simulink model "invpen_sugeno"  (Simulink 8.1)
settings: Solver=ode5  SolverMode=SingleTasking  StartTime=0.0  StopTime=1000  FixedStep=.01  MaxStep=0.1  RelTol=1e-3  AbsTol=1e-6
PreLoadFcn:
  | init_s;
undefined symbols (not defined in the file or in its folder): g, init_cond, l, m, mc
libraries: fuzblock x1

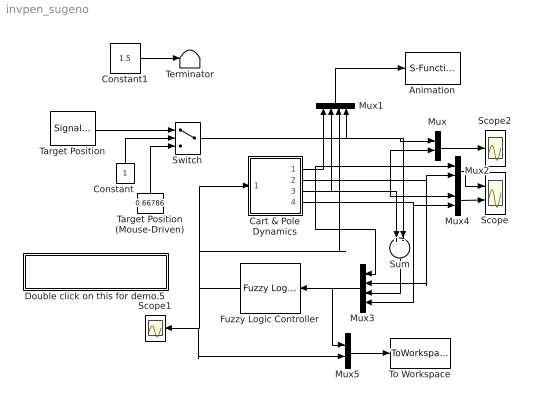
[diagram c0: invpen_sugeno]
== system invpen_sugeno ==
  Animation : S-Function  FunctionName=animcp  EnableBusSupport=off
  Cart & Pole Dynamics : Subsystem
  Constant : Constant
  Constant1 : Constant  Value=1.5
  Double click on this for demo.5 : Subsystem
  Fuzzy Logic Controller : fuzblock/Fuzzy Logic  Controller  fis=fismatrix
  Mux{,2,4..5} (4 alike) : Mux  Inputs=2
  Mux1 : Mux
  Mux3 : Mux
  Scope : Scope  NumInputPorts=2
  Scope1 : Scope
  Scope2 : Scope
  Sum : Sum  Inputs=+-
  Switch : Switch
  Target Position : SignalGenerator  WaveForm=square  Amplitude=1.500000  Frequency=0.628320  Units=rad/sec
  Target Position (Mouse-Driven) : Constant  Value=0.66786
  Terminator : Terminator
  To Workspace : ToWorkspace  VariableName=dataset  SampleTime=-1
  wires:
  Target Position/1 -> Switch/1
  Constant/1 -> Switch/2
  Target Position (Mouse-Driven)/1 -> Switch/3
  Mux1/1 -> Animation/1
  Cart & Pole Dynamics/4(out_4) -> Mux4/2, Mux3/4
  Sum/1 -> Mux3/3
  Mux3/1 -> Mux5/1, Fuzzy Logic Controller/1
  Mux/1 -> Scope2/1
  Mux2/1 -> Scope/1
  Mux4/1 -> Scope/2
  Cart & Pole Dynamics/3(out_3) -> Sum/1, Mux4/1, Mux/2, Mux1/2
  Cart & Pole Dynamics/1(out_1) -> Mux2/1, Mux3/1, Mux1/1
  Cart & Pole Dynamics/2(out_2) -> Mux2/2, Mux3/2
  Switch/1 -> Mux1/4, Sum/2, Mux/1
  Fuzzy Logic Controller/1 -> Mux5/2, Scope1/1, Mux1/3, Cart & Pole Dynamics/1(in_1)
  Constant1/1 -> Terminator/1
  Mux5/1 -> To Workspace/1

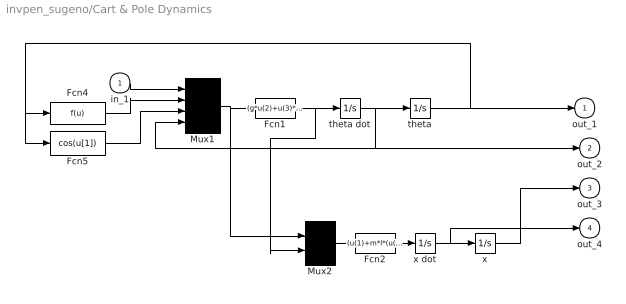
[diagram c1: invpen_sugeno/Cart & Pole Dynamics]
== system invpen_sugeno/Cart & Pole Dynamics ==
  in_1 : Inport
  Fcn1 : Fcn  Expr=(g*u(2)+u(3)*((-u(1)-m*l*u(4)*u(4)*u(2))/(mc+m)))/(l*(4/3-(m*u(3)*u(3))/(mc+m)))
  Fcn2 : Fcn  Expr=(u(1)+m*l*(u(4)*u(4)*u(2)-u(5)*u(3)))/(mc+m)
  Fcn4 : Fcn
  Fcn5 : Fcn  Expr=cos(u[1])
  Mux1 : Mux
  Mux2 : Mux  Inputs=[4,1]
  theta : Integrator  InitialCondition=init_cond(1)
  theta dot : Integrator  InitialCondition=init_cond(2)
  x : Integrator  InitialCondition=init_cond(3)
  x dot : Integrator  InitialCondition=init_cond(4)
  out_1 : Outport  InitialOutput=0
  out_2 : Outport  Port=2  InitialOutput=0
  out_3 : Outport  Port=3  InitialOutput=0
  out_4 : Outport  Port=4  InitialOutput=0
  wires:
  in_1/1 -> Mux1/1
  x/1 -> out_3/1
  x dot/1 -> out_4/1, x/1
  Mux1/1 -> Fcn1/1, Mux2/1
  Mux2/1 -> Fcn2/1
  Fcn2/1 -> x dot/1
  Fcn1/1 -> Mux2/2, theta dot/1
  theta dot/1 -> Mux1/4, out_2/1, theta/1
  Fcn4/1 -> Mux1/2
  Fcn5/1 -> Mux1/3
  theta/1 -> Fcn4/1, Fcn5/1, out_1/1

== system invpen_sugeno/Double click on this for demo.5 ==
